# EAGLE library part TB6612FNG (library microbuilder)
TB6612FNG Dual H-Bridge Motor Driver
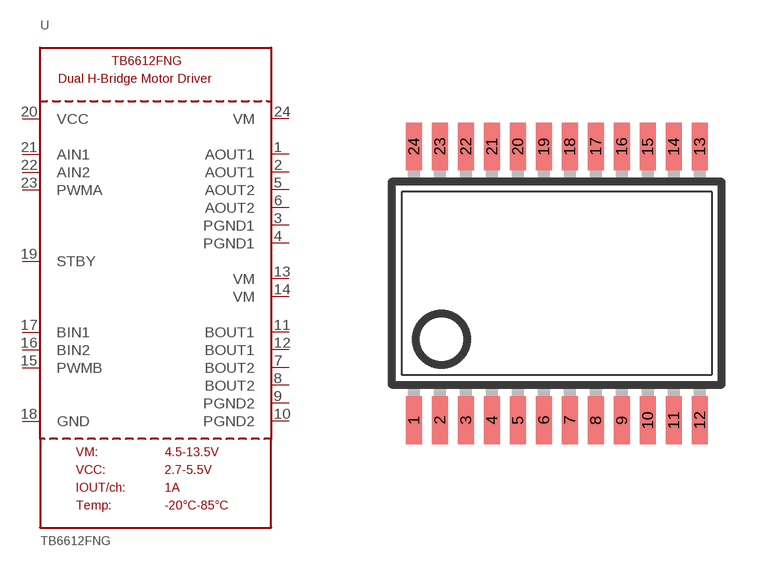
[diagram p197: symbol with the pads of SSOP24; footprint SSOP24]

Designator prefix U

## TB6612FNGSSOP  [SSOP24]
1  AOUT1  out
2  AOUT1  out
3  PGND1  pwr
4  PGND1  pwr
5  AOUT2  out
6  AOUT2  out
7  BOUT2  out
8  BOUT2  out
9  PGND2  pwr
10  PGND2  pwr
11  BOUT1  out
12  BOUT1  out
13  VM  pwr
14  VM  pwr
15  PWMB  in
16  BIN2  in
17  BIN1  in
18  GND  pwr
19  STBY  in
20  VCC  pwr
21  AIN1  in
22  AIN2  in
23  PWMA  in
24  VM  pwr

## Footprint SSOP24 (pad centres in mm)
Small Shrink Outline Package SOT340-1 / JEDEC MO-150AG
smd 0.4 x 1.2: 1 -3.575,-3.42; 2 -2.925,-3.42; 3 -2.275,-3.42; 4 -1.625,-3.42; 5 -0.975,-3.42; 6 -0.325,-3.42; 7 0.325,-3.42; 8 0.975,-3.42; 9 1.625,-3.42; 10 2.275,-3.42; 11 2.925,-3.42; 12 3.575,-3.42; 13 3.575,3.42; 14 2.925,3.42; 15 2.275,3.42; 16 1.625,3.42; 17 0.975,3.42; 18 0.325,3.42; 19 -0.325,3.42; 20 -0.975,3.42; 21 -1.625,3.42; 22 -2.275,3.42; 23 -2.925,3.42; 24 -3.575,3.42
